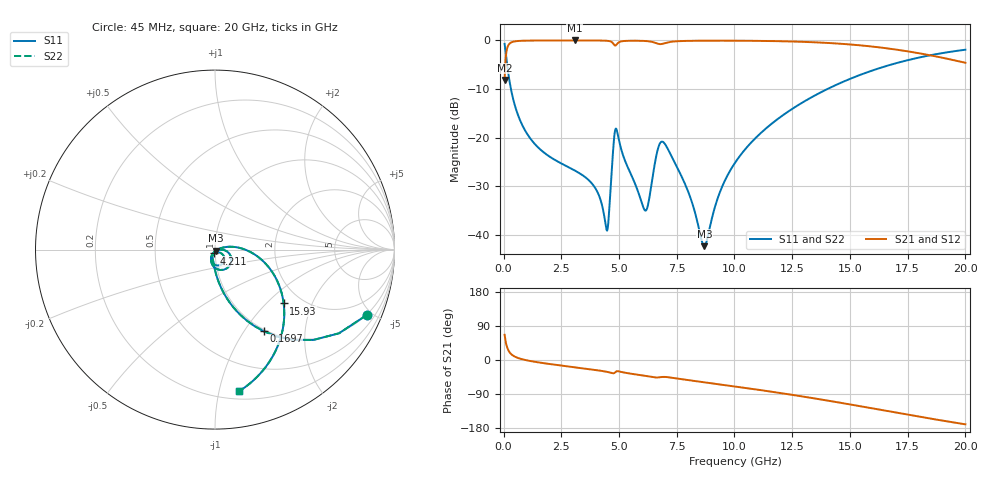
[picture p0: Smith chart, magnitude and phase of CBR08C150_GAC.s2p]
! S-parameter model data by Modelithics Inc.  support@modelithics.com 813-866-6335  Tampa FL USA
! S-Parameter data specifications:
! Substrate: 20-mil Rogers 4350B, substrate thickness, H=0.508mm, Dielectric constant, Er=3.75
! PCB Mounting Pad Footprint: Pad width, PadW=1.45mm , Pad length, PadL=1mm , Pad gap, PadG (edge-to-edge)=0.6mm , Reference planes=2.6mm apart
#  GHz  S  MA  R 50
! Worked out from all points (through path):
!   801 points, 45 MHz to 20 GHz, reference 50 ohm
!   highest |S21| = -0.02 dB at 3.088 GHz (marker M1); lowest = -8.1 dB at 45 MHz (marker M2)
!   group delay of S21, straight-line fit = 24.5 ps
!   lowest |S11| = -42.4 dB at 8.7 GHz (marker M3), VSWR 1.02, Z = 50.5 - j0.608 ohm
!   |S11| at or under -10 dB: 318.6 MHz to 14.03 GHz (13.71 GHz wide, 191 % of centre)
!   |S22| runs from -42.4 to -0.7 dB; largest |S21 - S12| = 0
!   S11 on the Smith chart (normalised r, x): 45 MHz: 0.97, -4.63; 169.7 MHz: 0.97, -1.23; 4.211 GHz: 0.99, -0.04; 15.93 GHz: 1.62, -1.27; 20 GHz: 0.26, -1.15
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0.045  0.9199 -23.4  0.3919 66.6  0.3919 66.6  0.9199 -23.4
0.169719  0.5288 -59.3  0.8484 30.7  0.8484 30.7  0.5288 -59.3
0.394213  0.2609 -77.6  0.9648 12.3  0.9648 12.3  0.2609 -77.6
1.04275  0.107 -90.9  0.9934 -1.3  0.9934 -1.3  0.107 -90.9
3.088138  0.04572 -107.6  0.9972 -19.3  0.9972 -19.3  0.04572 -107.6
3.387462  0.04144 -109.5  0.9972 -21.6  0.9972 -21.6  0.04144 -109.5
4.210606  0.02239 -108.2  0.9953 -28.4  0.9953 -28.4  0.02239 -108.2
4.410156  0.01303 -86.5  0.9922 -30.4  0.9922 -30.4  0.01303 -86.5
4.509931  0.01159 -40.3  0.988 -31.6  0.988 -31.6  0.01159 -40.3
4.759369  0.08257 -15.4  0.9213 -35.0  0.9213 -35.0  0.08257 -15.4
4.884087  0.1222 -66.8  0.8987 -30.1  0.8987 -30.1  0.1222 -66.8
6.131275  0.01771 -76.2  0.9846 -42.0  0.9846 -42.0  0.01771 -76.2
6.704981  0.07949 -49.9  0.9199 -46.0  0.9199 -46.0  0.07949 -49.9
6.979362  0.08634 -88.0  0.9347 -44.7  0.9347 -44.7  0.08634 -88.0
7.677787  0.0412 -118.4  0.9831 -50.3  0.9831 -50.3  0.0412 -118.4
8.700481  0.00762 -52.2  0.9915 -58.9  0.9915 -58.9  0.00762 -52.2
9.349019  0.02664 11.8  0.9922 -64.2  0.9922 -64.2  0.02664 11.8
10.0225  0.05494 13.9  0.9915 -69.8  0.9915 -69.8  0.05494 13.9
13.36496  0.2617 -11.8  0.9573 -100.4  0.9573 -100.4  0.2617 -11.8
15.93417  0.4861 -38.1  0.8646 -127.2  0.8646 -127.2  0.4861 -38.1
16.68248  0.5539 -46.1  0.8229 -135.3  0.8229 -135.3  0.5539 -46.1
20  0.8007 -80.4  0.5876 -169.8  0.5876 -169.8  0.8007 -80.4
